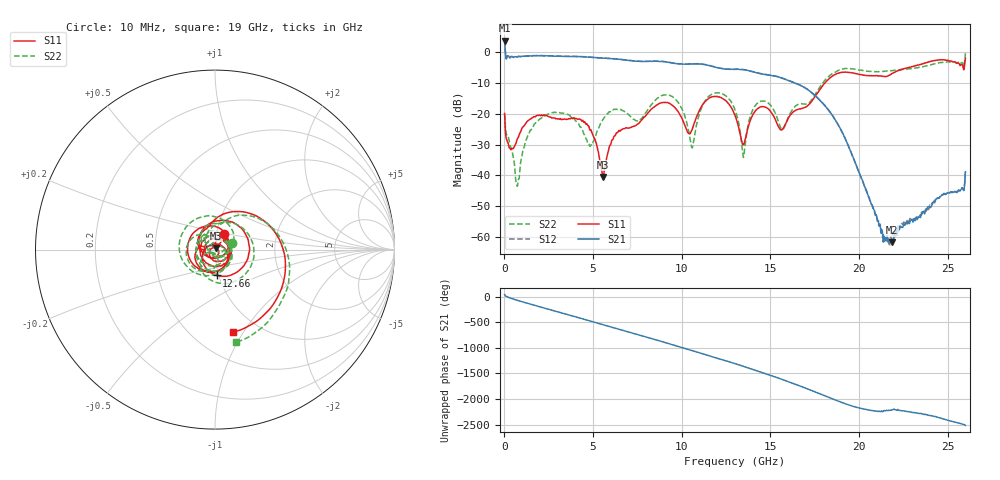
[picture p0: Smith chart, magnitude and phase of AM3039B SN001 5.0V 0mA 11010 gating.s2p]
!Agilent Technologies,E8364B,MY43040894,A.07.50.67
!Agilent E8364B: A.07.50.67
!Date: Tuesday, June 28, 2016 08:12:21
!Correction: S11(Full 2 Port(1,2))
!S21(Full 2 Port(1,2))
!S12(Full 2 Port(1,2))
!S22(Full 2 Port(1,2))
!S2P File: Measurements: S11, S21, S12, S22:
# Hz S  dB  R 50
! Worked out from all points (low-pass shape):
!   1601 points, 10 MHz to 26 GHz, reference 50 ohm
!   highest |S21| = 3.80 dB at 10 MHz (marker M1); lowest = -61.7 dB at 21.86 GHz (marker M2)
!   |S21| within 3 dB of the highest: start of sweep to 43.88 MHz
!   lowest |S11| = -40.4 dB at 5.565 GHz (marker M3), VSWR 1.02, Z = 50.3 + j0.91 ohm
!   |S11| at or under -10 dB: start of sweep to 18.07 GHz
!   |S22| runs from -43.5 to -0.3 dB; largest |S21 - S12| = 0.023
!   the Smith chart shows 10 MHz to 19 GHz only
!   S11 on the Smith chart (normalised r, x): 10 MHz: 1.09, +0.19; 12.66 GHz: 0.98, -0.29; 19 GHz: 0.76, -0.90
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1e7  -19.85 59.3  3.80 41.0  3.85 41.7  -19.99 20.1
7.572125e8  -27.91 84.3  -1.41 -74.2  -1.36 -74.0  -42.52 22.7
1.748081e9  -20.90 -5.8  -1.14 -174.1  -1.09 -173.8  -23.03 -33.9
2.820169e9  -21.31 -154.7  -1.22 81.0  -1.17 81.1  -19.41 -177.8
4.347081e9  -22.22 -34.5  -1.42 -67.9  -1.39 -67.7  -24.71 -42.2
5.565362e9  -40.44 72.1  -1.91 171.6  -1.85 171.7  -21.80 18.9
7.238469e9  -24.09 93.9  -2.81 5.5  -2.76 5.6  -21.58 116.1
8.684162e9  -16.77 -141.5  -2.90 -138.2  -2.85 -138.1  -14.70 -152.1
9.837469e9  -19.60 52.7  -3.76 104.0  -3.71 103.9  -16.62 51.8
1.084458e10  -20.88 165.3  -3.74 0.9  -3.69 0.7  -23.31 143.5
1.266388e10  -16.83 -86.6  -5.50 168.2  -5.46 167.9  -15.15 -95.0
1.3005e10  -20.47 -135.6  -5.52 132.0  -5.48 131.7  -18.70 -133.8
1.40446e10  -19.93 -53.3  -6.36 13.0  -6.32 12.6  -18.29 -105.3
1.558776e10  -25.14 170.9  -8.23 -168.0  -8.18 -168.4  -24.56 125.0
1.734208e10  -15.79 92.4  -13.14 -36.9  -13.13 -37.5  -15.37 70.4
1.899894e10  -6.54 -77.8  -25.35 95.8  -25.38 95.0  -5.52 -77.5
2.007103e10  -7.20 170.2  -40.00 -21.5  -40.07 -21.2  -5.77 178.7
2.167916e10  -7.49 45.8  -60.92 -58.8  -62.25 -64.3  -6.05 52.3
2.185784e10  -6.89 33.4  -61.70 -56.1  -60.51 -44.7  -5.94 38.6
2.348222e10  -3.91 -94.0  -53.39 -121.5  -53.01 -128.7  -4.80 -83.3
2.457055e10  -2.43 175.4  -46.84 149.2  -46.94 149.7  -3.34 -167.4
2.6e10  -1.86 7.7  -38.78 2.6  -38.72 1.1  -0.32 41.5
